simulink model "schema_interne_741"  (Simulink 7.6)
settings: Solver=ode15s  StartTime=0.0  StopTime=2.0  RelTol=1e-3
InitFcn:
  | clc
  | clear all
StopFcn:
  | close all, clc
  | load signaux.mat
  | plot(x(1,:),x(2,:),x(1,:),x(3,:),x(1,:),x(4,:))
  | title('Entrée & Sorties du schéma interne et Aop Simscape')
  | axis([0 2 -2.5 2.5])
  | xlabel('temps')
  | grid
libraries: fl_lib x25, elec_lib x23, nesl_utility x4

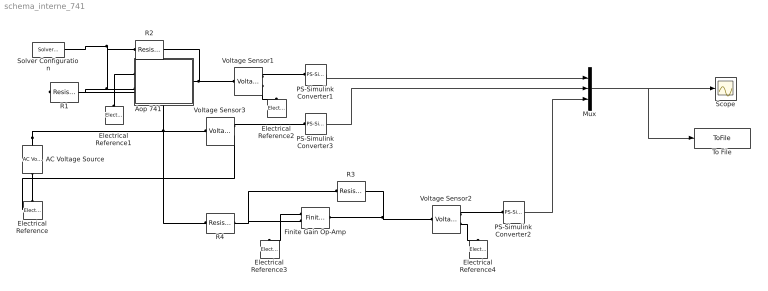
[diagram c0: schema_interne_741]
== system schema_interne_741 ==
  AC Voltage Source : fl_lib/Electrical/Electrical Sources/AC Voltage Source  DialogController=NetworkEngine.DynNeDlgSource  SystemSampleTime=-1  amp=1 V  shift=0 rad  omega=1 Hz  i_Log=off  v_Log=off  LocalVarNames=|current|voltage|power  LocalVarDescs=|Current (A)|Voltage (V)|Power (W)  LocalVarLogging=[0 0 0]
  Aop 741 : Subsystem
  Electrical Reference{,1..4} (5 alike) : fl_lib/Electrical/Electrical Elements/Electrical Reference  DialogController=NetworkEngine.DynNeDlgSource  SystemSampleTime=-1  i_Log=off  LocalVarNames=|i  LocalVarDescs=|i  LocalVarLogging=[]
  Finite Gain Op-Amp : elec_lib/Integrated Circuits/Finite Gain Op-Amp  DialogController=NetworkEngine.DynNeDlgSource  SystemSampleTime=-1  A=1000  Rin=1e+6 Ohm  Rout=100 Ohm  Vmin=-15 V  Vmax=15 V  LocalVarLogging=[]
  Mux : Mux  Inputs=3
  PS-Simulink Converter1 : nesl_utility/PS-Simulink Converter  DialogController=NetworkEngine.DynNeUtilDlgSource  SystemSampleTime=-1  PhysicalDomain=network_engine_domain  LeftPortType=input  RightPortType=output  SubClassName=ps_output  Unit=1  AffineConversion=off
  PS-Simulink Converter2 : nesl_utility/PS-Simulink Converter  DialogController=NetworkEngine.DynNeUtilDlgSource  SystemSampleTime=-1  PhysicalDomain=network_engine_domain  LeftPortType=input  RightPortType=output  SubClassName=ps_output  Unit=1  AffineConversion=off
  PS-Simulink Converter3 : nesl_utility/PS-Simulink Converter  DialogController=NetworkEngine.DynNeUtilDlgSource  SystemSampleTime=-1  PhysicalDomain=network_engine_domain  LeftPortType=input  RightPortType=output  SubClassName=ps_output  Unit=1  AffineConversion=off
  R1 : fl_lib/Electrical/Electrical Elements/Resistor  DialogController=NetworkEngine.DynNeDlgSource  SystemSampleTime=-1  R=10 kOhm  i_Log=off  v_Log=off  LocalVarNames=|current|voltage|power  LocalVarDescs=|Resistor current (A)|Voltage across resistor (V)|Power (W)  LocalVarLogging=[0 0 0]
  R2 : fl_lib/Electrical/Electrical Elements/Resistor  DialogController=NetworkEngine.DynNeDlgSource  SystemSampleTime=-1  R=22 kOhm  i_Log=off  v_Log=off  LocalVarNames=|current|voltage|power  LocalVarDescs=|Resistor current (A)|Voltage across resistor (V)|Power (W)  LocalVarLogging=[0 0 0]
  R3 : fl_lib/Electrical/Electrical Elements/Resistor  DialogController=NetworkEngine.DynNeDlgSource  SystemSampleTime=-1  R=22 kOhm  i_Log=off  v_Log=off  LocalVarNames=|current|voltage|power  LocalVarDescs=|Resistor current (A)|Voltage across resistor (V)|Power (W)  LocalVarLogging=[0 0 0]
  R4 : fl_lib/Electrical/Electrical Elements/Resistor  DialogController=NetworkEngine.DynNeDlgSource  SystemSampleTime=-1  R=10 kOhm  i_Log=off  v_Log=off  LocalVarNames=|current|voltage|power  LocalVarDescs=|Resistor current (A)|Voltage across resistor (V)|Power (W)  LocalVarLogging=[0 0 0]
  Scope : Scope
  Solver Configuration : nesl_utility/Solver Configuration  DialogController=NetworkEngine.DynNeUtilDlgSource  SystemSampleTime=-1  PhysicalDomain=network_engine_domain  LeftPortType=input  RightPortType=generic  SubClassName=solver  Accelerate=off  Profile=off  ResidualTolerance=1e-9  MaxNonlinIter=12  MaxModeIter=2  DoFixedCost=off  UseLocalSampling=off  DoDC=off  LinearAlgebra=Sparse  LocalSolverSampleTime=.001  LocalSolverChoice=NE_BACKWARD_EULER_ADVANCER  UseLocalSolver=off
  To File : ToFile  Filename=signaux  MatrixName=x
  Voltage Sensor1 : fl_lib/Electrical/Electrical Sensors/Voltage Sensor  DialogController=NetworkEngine.DynNeDlgSource  SystemSampleTime=-1  i1_Log=off  v1_Log=off  LocalVarNames=|i1|v1  LocalVarDescs=|i1|v1  LocalVarLogging=[]
  Voltage Sensor2 : fl_lib/Electrical/Electrical Sensors/Voltage Sensor  DialogController=NetworkEngine.DynNeDlgSource  SystemSampleTime=-1  i1_Log=off  v1_Log=off  LocalVarNames=|i1|v1  LocalVarDescs=|i1|v1  LocalVarLogging=[]
  Voltage Sensor3 : fl_lib/Electrical/Electrical Sensors/Voltage Sensor  DialogController=NetworkEngine.DynNeDlgSource  SystemSampleTime=-1  i1_Log=off  v1_Log=off  LocalVarNames=|i1|v1  LocalVarDescs=|i1|v1  LocalVarLogging=[]
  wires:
  PS-Simulink Converter1/1 -> Mux/1
  Mux/1 -> Scope/1, To File/1
  PS-Simulink Converter3/1 -> Mux/2
  PS-Simulink Converter2/1 -> Mux/3
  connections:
  Electrical Reference/LConn1 -- AC Voltage Source/RConn1 -- Voltage Sensor3/RConn2
  AC Voltage Source/LConn1 -- R1/LConn1 -- Voltage Sensor3/LConn1 -- R4/LConn1
  Aop 741/RConn1 -- Voltage Sensor1/LConn1 -- R2/RConn1
  Voltage Sensor1/RConn2 -- Electrical Reference2/LConn1
  Voltage Sensor1/RConn1 -- PS-Simulink Converter1/LConn1
  Electrical Reference1/LConn1 -- Aop 741/LConn1
  Aop 741/LConn2 -- R2/LConn1 -- Solver Configuration/RConn1 -- R1/RConn1
  Voltage Sensor3/RConn1 -- PS-Simulink Converter3/LConn1
  Voltage Sensor2/RConn1 -- PS-Simulink Converter2/LConn1
  R4/RConn1 -- Finite Gain Op-Amp/LConn2 -- R3/LConn1
  Finite Gain Op-Amp/LConn1 -- Electrical Reference3/LConn1
  Finite Gain Op-Amp/RConn1 -- Voltage Sensor2/LConn1 -- R3/RConn1
  Voltage Sensor2/RConn2 -- Electrical Reference4/LConn1

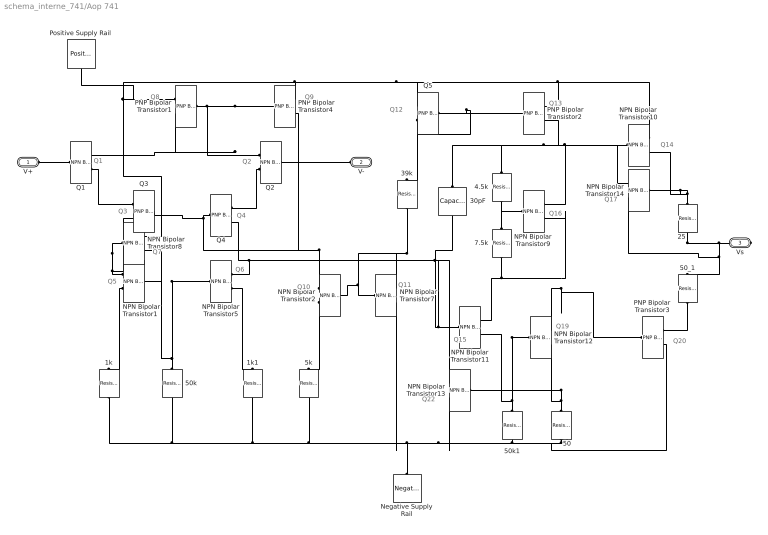
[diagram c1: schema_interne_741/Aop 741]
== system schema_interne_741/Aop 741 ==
  note: Q4
  note: Q3
  note: Q1
  note: Q2
  note: Q7
  note: Q6
  note: Q5
  note: Q8
  note: Q9
  note: Q10
  note: Q14
  note: Q17
  note: Q13
  note: Q16
  note: Q11
  note: Q12
  note: Q15
  note: Q22
  note: Q19
  note: Q20
  1k : fl_lib/Electrical/Electrical Elements/Resistor  DialogController=NetworkEngine.DynNeDlgSource  SystemSampleTime=-1  R=1 kOhm  i_Log=off  v_Log=off  LocalVarNames=|i|v  LocalVarDescs=|i|v  LocalVarLogging=[0 0]
  1k1 : fl_lib/Electrical/Electrical Elements/Resistor  DialogController=NetworkEngine.DynNeDlgSource  SystemSampleTime=-1  R=1 kOhm  i_Log=off  v_Log=off  LocalVarNames=|i|v  LocalVarDescs=|i|v  LocalVarLogging=[0 0]
  25 : fl_lib/Electrical/Electrical Elements/Resistor  DialogController=NetworkEngine.DynNeDlgSource  SystemSampleTime=-1  R=25 Ohm  i_Log=off  v_Log=off  LocalVarNames=|i|v  LocalVarDescs=|i|v  LocalVarLogging=[0 0]
  30pF : fl_lib/Electrical/Electrical Elements/Capacitor  DialogController=NetworkEngine.DynNeDlgSource  SystemSampleTime=-1  c=30 pF  v0=0 V  r=1e-6 Ohm  g=0 1/Ohm  i_Log=off  v_Log=off  vc_Log=off  LocalVarNames=|i|v|vc  LocalVarDescs=|i|v|Internal variable for voltage across capacitor term  LocalVarLogging=[0 0 0]
  39k : fl_lib/Electrical/Electrical Elements/Resistor  DialogController=NetworkEngine.DynNeDlgSource  SystemSampleTime=-1  R=39 kOhm  i_Log=off  v_Log=off  LocalVarNames=|i|v  LocalVarDescs=|i|v  LocalVarLogging=[0 0]
  4.5k : fl_lib/Electrical/Electrical Elements/Resistor  DialogController=NetworkEngine.DynNeDlgSource  SystemSampleTime=-1  R=4.5 kOhm  i_Log=off  v_Log=off  LocalVarNames=|i|v  LocalVarDescs=|i|v  LocalVarLogging=[0 0]
  50 : fl_lib/Electrical/Electrical Elements/Resistor  DialogController=NetworkEngine.DynNeDlgSource  SystemSampleTime=-1  R=50 Ohm  i_Log=off  v_Log=off  LocalVarNames=|i|v  LocalVarDescs=|i|v  LocalVarLogging=[0 0]
  50_1 : fl_lib/Electrical/Electrical Elements/Resistor  DialogController=NetworkEngine.DynNeDlgSource  SystemSampleTime=-1  R=50 Ohm  i_Log=off  v_Log=off  LocalVarNames=|i|v  LocalVarDescs=|i|v  LocalVarLogging=[0 0]
  50k : fl_lib/Electrical/Electrical Elements/Resistor  DialogController=NetworkEngine.DynNeDlgSource  SystemSampleTime=-1  R=50 kOhm  i_Log=off  v_Log=off  LocalVarNames=|i|v  LocalVarDescs=|i|v  LocalVarLogging=[0 0]
  50k1 : fl_lib/Electrical/Electrical Elements/Resistor  DialogController=NetworkEngine.DynNeDlgSource  SystemSampleTime=-1  R=50 kOhm  i_Log=off  v_Log=off  LocalVarNames=|i|v  LocalVarDescs=|i|v  LocalVarLogging=[0 0]
  5k : fl_lib/Electrical/Electrical Elements/Resistor  DialogController=NetworkEngine.DynNeDlgSource  SystemSampleTime=-1  R=5 kOhm  i_Log=off  v_Log=off  LocalVarNames=|i|v  LocalVarDescs=|i|v  LocalVarLogging=[0 0]
  7.5k : fl_lib/Electrical/Electrical Elements/Resistor  DialogController=NetworkEngine.DynNeDlgSource  SystemSampleTime=-1  R=7.5 kOhm  i_Log=off  v_Log=off  LocalVarNames=|i|v  LocalVarDescs=|i|v  LocalVarLogging=[0 0]
  NPN Bipolar Transistor{1..2,5,7..14} (11 alike) : elec_lib/Semiconductor Devices/NPN Bipolar Transistor  DialogController=NetworkEngine.DynNeDlgSource  SystemSampleTime=-1  parameterization=1  BF=100  IS=1e-14 A  VAF=200 V  hfe=100  hoe=5e-5 1/Ohm  Ic_h=1 mA  V1=0.55 V  I1=0.5 mA  BR=1  Tmeas=25 C  RC=0.01 Ohm  RE=1e-4 Ohm  RB=1 Ohm  C_BC=5 pF  C_BE=5 pF  TF=0 us  TR=0 us  LocalVarLogging=[]
  Negative Supply Rail : elec_lib/Sources/Negative Supply Rail  DialogController=NetworkEngine.DynNeDlgSource  SystemSampleTime=-1  v0=-15 V  current_Log=off  voltage_Log=off  power_Log=off  LocalVarNames=|current|voltage|power  LocalVarDescs=|Current (A)|Voltage (V)|Power (W)  LocalVarLogging=[0 0 0]
  PNP Bipolar Transistor{1..4} (4 alike) : elec_lib/Semiconductor Devices/PNP Bipolar Transistor  DialogController=NetworkEngine.DynNeDlgSource  SystemSampleTime=-1  parameterization=1  BF=100  IS=1e-14 A  VAF=200 V  hfe=100  hoe=5e-5 1/Ohm  Ic_h=1 mA  V1=0.55 V  I1=0.5 mA  BR=1  Tmeas=25 C  RC=0.01 Ohm  RE=1e-4 Ohm  RB=1 Ohm  C_BC=5 pF  C_BE=5 pF  TF=0 us  TR=0 us  LocalVarLogging=[]
  Positive Supply Rail : elec_lib/Sources/Positive Supply Rail  DialogController=NetworkEngine.DynNeDlgSource  SystemSampleTime=-1  v0=15 V  current_Log=off  voltage_Log=off  power_Log=off  LocalVarNames=|current|voltage|power  LocalVarDescs=|Current (A)|Voltage (V)|Power (W)  LocalVarLogging=[0 0 0]
  Q1 : elec_lib/Semiconductor Devices/NPN Bipolar Transistor  DialogController=NetworkEngine.DynNeDlgSource  SystemSampleTime=-1  parameterization=1  BF=100  IS=1e-14 A  VAF=200 V  hfe=100  hoe=5e-5 1/Ohm  Ic_h=1 mA  V1=0.55 V  I1=0.5 mA  BR=1  Tmeas=25 C  RC=0.01 Ohm  RE=1e-4 Ohm  RB=1 Ohm  C_BC=5 pF  C_BE=5 pF  TF=0 us  TR=0 us  LocalVarLogging=[]
  Q2 : elec_lib/Semiconductor Devices/NPN Bipolar Transistor  DialogController=NetworkEngine.DynNeDlgSource  SystemSampleTime=-1  parameterization=1  BF=100  IS=1e-14 A  VAF=200 V  hfe=100  hoe=5e-5 1/Ohm  Ic_h=1 mA  V1=0.55 V  I1=0.5 mA  BR=1  Tmeas=25 C  RC=0.01 Ohm  RE=1e-4 Ohm  RB=1 Ohm  C_BC=5 pF  C_BE=5 pF  TF=0 us  TR=0 us  LocalVarLogging=[]
  Q3 : elec_lib/Semiconductor Devices/PNP Bipolar Transistor  DialogController=NetworkEngine.DynNeDlgSource  SystemSampleTime=-1  parameterization=1  BF=100  IS=1e-14 A  VAF=200 V  hfe=100  hoe=5e-5 1/Ohm  Ic_h=1 mA  V1=0.55 V  I1=0.5 mA  BR=1  Tmeas=25 C  RC=0.01 Ohm  RE=1e-4 Ohm  RB=1 Ohm  C_BC=5 pF  C_BE=5 pF  TF=0 us  TR=0 us  LocalVarLogging=[]
  Q4 : elec_lib/Semiconductor Devices/PNP Bipolar Transistor  DialogController=NetworkEngine.DynNeDlgSource  SystemSampleTime=-1  parameterization=1  BF=100  IS=1e-14 A  VAF=200 V  hfe=100  hoe=5e-5 1/Ohm  Ic_h=1 mA  V1=0.55 V  I1=0.5 mA  BR=1  Tmeas=25 C  RC=0.01 Ohm  RE=1e-4 Ohm  RB=1 Ohm  C_BC=5 pF  C_BE=5 pF  TF=0 us  TR=0 us  LocalVarLogging=[]
  Q5 : elec_lib/Semiconductor Devices/PNP Bipolar Transistor  DialogController=NetworkEngine.DynNeDlgSource  SystemSampleTime=-1  parameterization=1  BF=100  IS=1e-14 A  VAF=200 V  hfe=100  hoe=5e-5 1/Ohm  Ic_h=1 mA  V1=0.55 V  I1=0.5 mA  BR=1  Tmeas=25 C  RC=0.01 Ohm  RE=1e-4 Ohm  RB=1 Ohm  C_BC=5 pF  C_BE=5 pF  TF=0 us  TR=0 us  LocalVarLogging=[]
  V+ : PMIOPort  Port=1  Side=Left
  V- : PMIOPort  Port=2  Side=Left
  Vs : PMIOPort  Port=3  Side=Right
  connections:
  NPN Bipolar Transistor1/RConn2 -- 1k/LConn1
  1k/RConn1 -- 50k/RConn1 -- 5k/RConn1 -- NPN Bipolar Transistor7/RConn2 -- NPN Bipolar Transistor13/RConn2 -- 50k1/RConn1 -- PNP Bipolar Transistor3/RConn2 -- 50/RConn1 -- Negative Supply Rail/LConn1 -- 1k1/RConn1
  NPN Bipolar Transistor5/RConn2 -- 1k1/LConn1
  NPN Bipolar Transistor9/LConn1 -- NPN Bipolar Transistor10/RConn2 -- NPN Bipolar Transistor14/LConn1
  Vs/RConn1 -- NPN Bipolar Transistor9/RConn1 -- 50_1/LConn1 -- NPN Bipolar Transistor14/RConn2
  39k/RConn1 -- NPN Bipolar Transistor7/RConn1 -- NPN Bipolar Transistor2/LConn1 -- NPN Bipolar Transistor7/LConn1
  PNP Bipolar Transistor2/RConn2 -- NPN Bipolar Transistor9/RConn1 -- NPN Bipolar Transistor10/LConn1 -- NPN Bipolar Transistor14/RConn1 -- 4.5k/LConn1 -- 30pF/LConn1
  4.5k/RConn1 -- 7.5k/LConn1 -- NPN Bipolar Transistor9/LConn1
  50/LConn1 -- NPN Bipolar Transistor12/RConn2 -- NPN Bipolar Transistor13/LConn1
  50_1/RConn1 -- PNP Bipolar Transistor3/RConn1
  50k/LConn1 -- NPN Bipolar Transistor1/LConn1 -- NPN Bipolar Transistor5/LConn1 -- NPN Bipolar Transistor8/RConn2
  50k1/LConn1 -- NPN Bipolar Transistor11/RConn2 -- NPN Bipolar Transistor12/LConn1
  NPN Bipolar Transistor2/RConn2 -- 5k/LConn1
  7.5k/RConn1 -- NPN Bipolar Transistor11/RConn1 -- NPN Bipolar Transistor9/RConn2 -- NPN Bipolar Transistor12/RConn1 -- PNP Bipolar Transistor3/LConn1
  NPN Bipolar Transistor1/RConn1 -- Q3/RConn2 -- NPN Bipolar Transistor8/LConn1
  NPN Bipolar Transistor10/RConn1 -- NPN Bipolar Transistor8/RConn1 -- PNP Bipolar Transistor1/RConn1 -- Positive Supply Rail/RConn1 -- PNP Bipolar Transistor4/RConn1 -- Q5/RConn1 -- PNP Bipolar Transistor2/RConn1
  NPN Bipolar Transistor2/RConn1 -- Q3/LConn1 -- Q4/LConn1 -- PNP Bipolar Transistor4/RConn2
  NPN Bipolar Transistor13/RConn1 -- NPN Bipolar Transistor11/LConn1 -- Q4/RConn2 -- NPN Bipolar Transistor5/RConn1 -- 30pF/RConn1
  PNP Bipolar Transistor1/LConn1 -- PNP Bipolar Transistor4/LConn1 -- Q1/RConn1 -- PNP Bipolar Transistor1/RConn2 -- Q2/RConn1
  Q5/RConn2 -- PNP Bipolar Transistor2/LConn1 -- Q5/LConn1 -- 39k/LConn1
  Q1/RConn2 -- Q3/RConn1
  Q2/RConn2 -- Q4/RConn1
  V+/RConn1 -- Q1/LConn1
  V-/RConn1 -- Q2/LConn1
